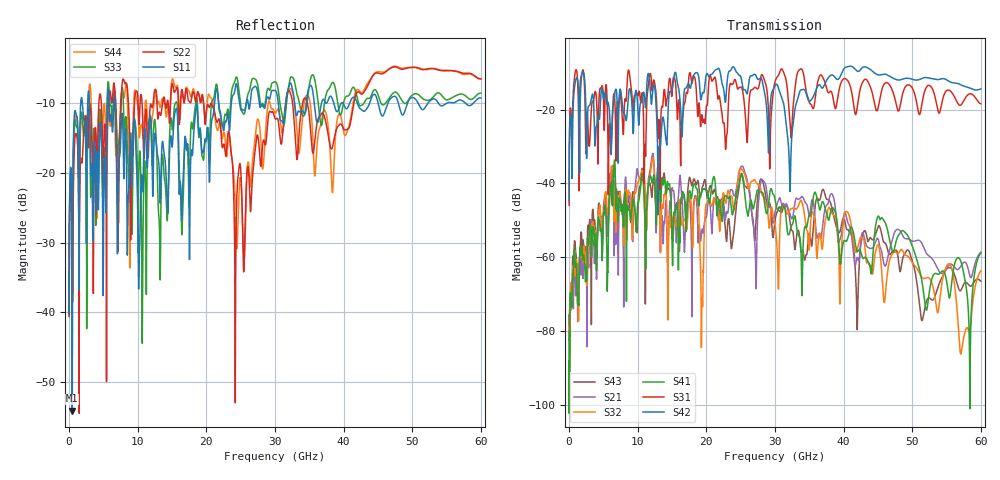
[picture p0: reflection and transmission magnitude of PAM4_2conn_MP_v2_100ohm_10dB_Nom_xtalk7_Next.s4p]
! Info: Touchstone file created by Circ.  Input file=FAB50GbE_2conn_Midplane_Examax_Topo2_v2_100ohm_10dB_Nom.circ
# Hz S RI R 50
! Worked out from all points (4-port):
!   6000 points, 10 MHz to 60 GHz, reference 50 ohm
!   strongest paths, dB at 10 MHz, 15.01 GHz, 30.01 GHz, 45.01 GHz, 60 GHz:
!     S42: -44.6, -14.5, -13.5, -10.6, -14.4
!     S31: -45.9, -15.7, -12.5, -19.7, -18.4
!     S41: -88.0, -57.2, -44.3, -48.9, -58.9
!     S32: -82.5, -49.7, -51.0, -56.6, -63.6
!     S21: -75.6, -41.2, -47.8, -55.0, -58.6
!     S43: -77.3, -54.8, -50.0, -51.8, -66.4
!   lowest |S11| = -54.1 dB at 470 MHz (marker M1), VSWR 1.00, Z = 49.8 + j0.0915 ohm
!   |S11| at or under -10 dB: 2.976 GHz to 5.571 GHz (2.595 GHz wide, 60.7 % of centre); 6.696 GHz to 21.2 GHz (14.51 GHz wide, 104 % of centre); 21.78 GHz to 23.64 GHz (1.852 GHz wide, 8.16 % of centre)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
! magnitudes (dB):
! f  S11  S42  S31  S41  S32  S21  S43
! 10 MHz  -40.1  -44.6  -45.9  -88.0  -82.5  -75.6  -77.3
! 470 MHz  -54.1  -32.0  -26.7  -67.6  -71.5  -68.4  -63.8
! 12.11 GHz  -18.5  -16.8  -15.0  -39.8  -33.6  -32.4  -42.9
! 19.35 GHz  -17.2  -16.0  -21.4  -42.2  -71.5  -52.6  -41.5
! 25.04 GHz  -11.0  -11.2  -13.9  -37.8  -35.9  -35.5  -37.7
! 32.15 GHz  -7.2  -39.0  -22.3  -53.3  -47.2  -48.1  -49.7
! 60 GHz  -9.3  -14.4  -18.4  -58.9  -63.6  -58.6  -66.4
